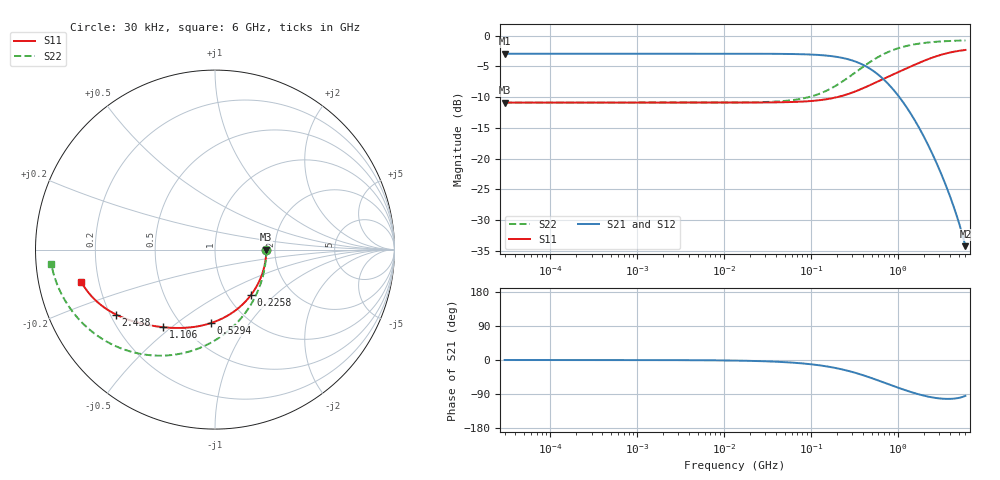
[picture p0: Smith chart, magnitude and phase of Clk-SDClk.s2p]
!EMIF06-MSD04F3
!Simulation
!24/03/11  09:02
!Start Freq. :30.000kHz; Stop Freq. : 6.000GHz
!Number of points : 1592; Sweep : LOGARITHMIC
!B1-B4 (Clk-SDClk)
!Freq ReS11 ImS11 ReS21 ImS21 ReS12 ImS12 ReS22 ImS22
# Hz  S  RI  R  50
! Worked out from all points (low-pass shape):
!   1592 points, 30 kHz to 6 GHz, reference 50 ohm
!   highest |S21| = -2.92 dB at 30 kHz (marker M1); lowest = -34.2 dB at 6 GHz (marker M2)
!   |S21| within 3 dB of the highest: start of sweep to 547 MHz
!   lowest |S11| = -10.9 dB at 30 kHz (marker M3), VSWR 1.80, Z = 90 - j0.00748 ohm
!   |S11| at or under -10 dB: start of sweep to 199.6 MHz
!   |S22| runs from -10.9 to -0.8 dB; largest |S21 - S12| = 1.4e-15
!   S11 on the Smith chart (normalised r, x): 30 kHz: 1.80, -0.00; 225.8 MHz: 1.27, -0.72; 529.4 MHz: 0.69, -0.68; 1.106 GHz: 0.39, -0.47; 2.438 GHz: 0.22, -0.29; 6 GHz: 0.13, -0.12
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30000  0.2857 -3.82e-05  0.7143 -4.23e-05  0.7143 -4.23e-05  0.2857 -6.1e-05
231093.6  0.2857 -0.000294  0.7143 -0.000326  0.7143 -0.000326  0.2857 -0.00047
1766531  0.2857 -0.00225  0.7143 -0.00249  0.7143 -0.00249  0.2857 -0.00359
1.350376e7  0.2854 -0.0172  0.7138 -0.019  0.7138 -0.019  0.2851 -0.0274
4.336319e7  0.2821 -0.0549  0.7096 -0.0608  0.7096 -0.0608  0.2792 -0.0877
6.820056e7  0.2768 -0.0858  0.7027 -0.0948  0.7027 -0.0948  0.2697 -0.1367
1.032257e8  0.2656 -0.1279  0.6883 -0.1408  0.6883 -0.1408  0.2496 -0.2034
1.586553e8  0.24 -0.1898  0.6553 -0.2073  0.6553 -0.2073  0.2038 -0.3001
2.258333e8  0.199 -0.2548  0.6029 -0.2745  0.6029 -0.2745  0.1307 -0.3987
2.778356e8  0.1625 -0.2968  0.5565 -0.3151  0.5565 -0.3151  0.066 -0.4595
3.39199e8  0.1167 -0.3369  0.4991 -0.3507  0.4991 -0.3507  -0.0143 -0.5141
4.303164e8  0.0485 -0.3799  0.4152 -0.3815  0.4152 -0.3815  -0.1322 -0.5648
5.294049e8  -0.0211 -0.4089  0.3326 -0.3922  0.3326 -0.3922  -0.2494 -0.5882
6.463304e8  -0.0935 -0.4272  0.251 -0.3849  0.251 -0.3849  -0.3668 -0.5879
7.890804e8  -0.1677 -0.4357  0.1743 -0.3606  0.1743 -0.3606  -0.4796 -0.5654
1.106084e9  -0.2898 -0.4322  0.0711 -0.2911  0.0711 -0.2911  -0.6411 -0.4893
1.598777e9  -0.416 -0.4104  0.00665 -0.2007  0.00665 -0.2007  -0.7633 -0.3828
2.438492e9  -0.5515 -0.3617  -0.0165 -0.1125  -0.0165 -0.1125  -0.8457 -0.2658
3.141386e9  -0.6229 -0.3183  -0.0156 -0.0744  -0.0156 -0.0744  -0.8752 -0.2046
3.985241e9  -0.6786 -0.2698  -0.0108 -0.0484  -0.0108 -0.0484  -0.8938 -0.1536
4.791313e9  -0.7131 -0.2294  -0.00643 -0.0334  -0.00643 -0.0334  -0.9038 -0.1179
6e9  -0.7451 -0.1795  -0.00153 -0.0193  -0.00153 -0.0193  -0.9121 -0.0778
